TYPE CHAMBER_OUT :
STRUCT
	//C07	EL2889 16DO
	C07		:ARRAY [1..16] OF BOOL;
	
	
	//C08	EL2889	16DO
	C08		:ARRAY [1..16] OF BOOL;
	
	
	//C09	EL2889	16DO
	C09		:ARRAY [1..16] OF BOOL;
	
	//C14	EL2904	4SDO
	C14		:ARRAY [1..4] OF BOOL;
END_STRUCT
END_TYPE
